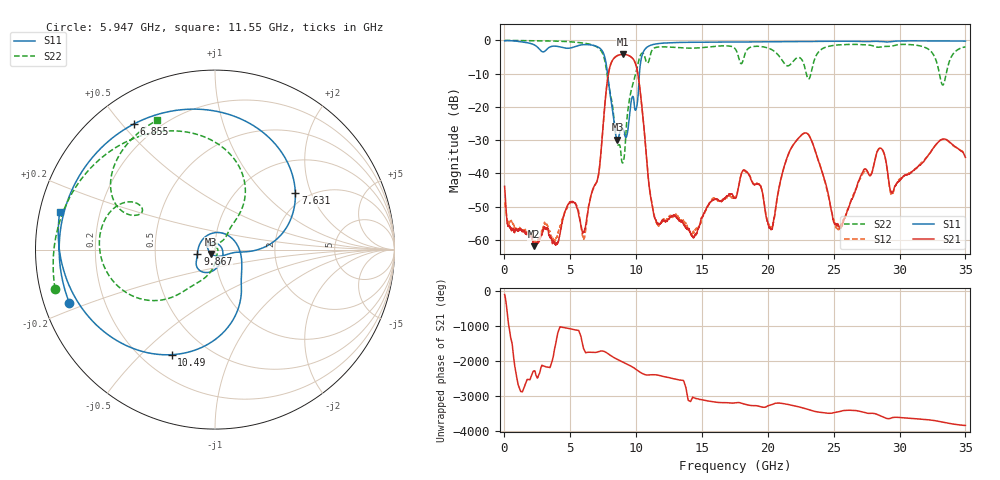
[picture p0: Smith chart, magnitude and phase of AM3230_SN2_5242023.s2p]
!Keysight Technologies,N5245B,MY58422270,A.16.20.02
!Date: Thursday, May 25, 2023 04:41:41
!Correction: S11(C  2-Port  )
!S21(C  2-Port  )
!S12(C  2-Port  )
!S22(C  2-Port  )
!S2P File: Measurements: S11, S21, S12, S22:
# Hz S  dB  R 50
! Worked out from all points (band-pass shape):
!   6401 points, 10 MHz to 35 GHz, reference 50 ohm
!   highest |S21| = -4.17 dB at 9.02 GHz (marker M1); lowest = -61.9 dB at 2.257 GHz (marker M2)
!   |S21| within 3 dB of the highest: 8.063 GHz to 9.966 GHz (1.903 GHz wide, 21.1 % of centre)
!   lowest |S11| = -29.8 dB at 8.577 GHz (marker M3), VSWR 1.07, Z = 47.9 - j2.34 ohm
!   |S11| at or under -10 dB: 7.828 GHz to 10.24 GHz (2.416 GHz wide, 26.7 % of centre)
!   |S22| runs from -36.8 to 0.0 dB; largest |S21 - S12| = 0.0051
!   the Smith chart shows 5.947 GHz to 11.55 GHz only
!   S11 on the Smith chart (normalised r, x): 5.947 GHz: 0.08, -0.18; 6.855 GHz: 0.12, +0.54; 7.631 GHz: 1.74, +1.56; 9.867 GHz: 0.82, -0.04; 10.49 GHz: 0.32, -0.62; 11.55 GHz: 0.06, +0.12
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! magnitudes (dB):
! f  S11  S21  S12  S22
! 10 MHz  -0.1  -43.9  -48.7  0.0
! 2.257 GHz  -1.3  -61.9  -60.6  -0.1
! 5.843 GHz  -1.3  -56.2  -56.8  -0.7
! 5.947 GHz  -1.3  -57.8  -58.9  -0.7
! 6.855 GHz  -1.6  -43.5  -43.6  -1.6
! 7.631 GHz  -5.2  -18.9  -18.9  -6.3
! 8.577 GHz  -29.8  -4.6  -4.6  -31.2
! 9.02 GHz  -26.8  -4.2  -4.2  -36.5
! 9.867 GHz  -20.0  -6.2  -6.2  -11.5
! 10.49 GHz  -4.0  -22.1  -22.1  -3.8
! 11.55 GHz  -1.0  -54.6  -55.0  -2.1
! 11.68 GHz  -0.9  -55.2  -55.6  -2.0
! 17.5 GHz  -0.5  -47.4  -47.1  -2.4
! 18.36 GHz  -0.5  -39.3  -39.7  -3.1
! 20.23 GHz  -0.4  -56.8  -56.1  -2.6
! 21.67 GHz  -0.4  -33.2  -33.3  -7.4
! 23.34 GHz  -0.3  -30.3  -30.3  -8.7
! 25.31 GHz  -0.2  -55.1  -56.8  -1.3
! 28.44 GHz  -0.3  -32.5  -32.5  -2.0
! 29.17 GHz  -0.4  -42.0  -42.4  -1.8
! 33.28 GHz  -0.2  -29.7  -29.7  -13.4
! 35 GHz  -0.2  -35.2  -34.0  -1.9
